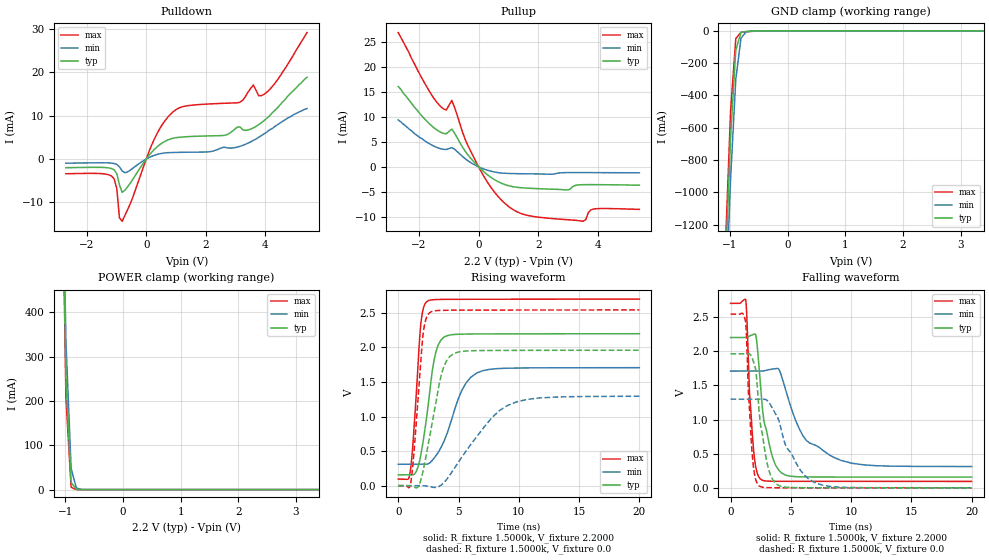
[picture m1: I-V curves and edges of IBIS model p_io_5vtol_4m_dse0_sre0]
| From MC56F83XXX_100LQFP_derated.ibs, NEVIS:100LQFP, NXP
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[Model] p_io_5vtol_4m_dse0_sre0
|   Model p_io_5vtol_4m_dse0_sre0
| Library cells for typ/min/max conditions are connected as defined below:
|  pad - External Pad
|  ipp_do - Core Input
|  ipp_obe - Output Buffer Enable
|  esd_boost - vdd_s_3v
|  esd_bus - vdd_s_3v
|  ipp_ame - vss_s_lv
|  ipp_dse - vss_s_lv
|  ipp_ina40a_5vtol - NC
|  ipp_ina40b_5vtol - NC
|  ipp_ina_5vtol - NC
|  ipp_ina_mux_3v - NC
|  ipp_ind - NC
|  ipp_ind_3v - NC
|  ipp_pue - vss_s_lv
|  ipp_sre - vss_s_lv
|  tie_3v - vdd_s_3v
|  tie_hi - vdd_s_lv
|  vbuf_3v - vdd_s_3v
|  vdd_bulk_lv - vdd_s_lv
|  vdd_s_3v - vdd_s_3v
|  vdd_s_lv - vdd_s_lv
|  vss_bulk - vss_s_3v
|  vss_s_3v - vss_s_3v
|  vss_s_lv - vss_s_lv
| All other pins connected to ground
Model_type I/O
Polarity   Non-Inverting
Enable   Active-High
Vinl =   0.7700V
Vinh =   1.5400V
Vmeas =  1.1000V
Cref =   25.0000pF
Rref =   1.0000k
Vref =   0.0V
C_comp   2.5897pF   2.5141pF   2.6932pF
[Temperature Range]   25.0000   0.1250k   -40.0000
[Voltage Range]   2.2000V   1.7100V   2.7000V
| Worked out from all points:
|   slope of the pulldown table from 0 to 0.33 V, typ, clamps not added: 128 ohm
|   slope of the pullup table from 0 to 0.33 V, typ, clamps not added: 190 ohm
|   GND clamp passes 1 mA (typ) near -0.56 V on its own axis
|   POWER clamp passes 1 mA (typ) near -0.81 V on its own axis
|   rising waveform, R_fixture 1.5000k, V_fixture 2.2000: 20-80 % time 947ps typ, 1.78ns min, 566ps max; typ from 0.156 V to 2.2 V
|   rising waveform, R_fixture 1.5000k, V_fixture 0.0: 20-80 % time 1.26ns typ, 3.4ns min, 656ps max; typ from 0 V to 1.96 V
|   falling waveform, R_fixture 1.5000k, V_fixture 2.2000: 20-80 % time 953ps typ, 2.78ns min, 464ps max; typ from 2.2 V to 0.158 V
|   falling waveform, R_fixture 1.5000k, V_fixture 0.0: 20-80 % time 819ps typ, 1.91ns min, 430ps max; typ from 1.96 V to 0.001 V
[Pulldown]
|Voltage   I(typ)   I(min)   I(max)
-2.7V     -2mA       -960uA     -3.39mA
-1.17V    -2.19mA    -943uA     -3.913mA
-990mV    -3.359mA   -1.244mA   -6.804mA
-900mV    -5.941mA   -1.821mA   -13.58mA
-810mV    -7.677mA   -2.75mA    -14.34mA
270mV     2.201mA    843.7uA    4.568mA
810mV     4.605mA    1.475mA    10.28mA
3.15V     7.385mA    2.91mA     13.07mA
3.6V      7.17mA     4.3mA      17.03mA
3.78V     7.91mA     5mA        14.56mA
3.96V     8.86mA     5.8mA      14.91mA
5.4V      18.8mA     11.6mA     29.1mA
[Pullup]
|Voltage   I(typ)   I(min)   I(max)
-2.7V     16.1mA     9.4mA      26.9mA
-1.44V    7.55mA     3.98mA     13.23mA
-1.08V    6.637mA    3.488mA    11.41mA
-900mV    7.558mA    3.848mA    13.31mA
-450mV    3.121mA    1.623mA    5.492mA
90mV      -525.5uA   -231.9uA   -998.2uA
540mV     -2.585mA   -1.04mA    -5.11mA
1.08V     -3.888mA   -1.337mA   -8.259mA
2.97V     -4.634mA   -1.154mA   -10.59mA
3.51V     -3.575mA   -1.148mA   -10.91mA
3.87V     -3.565mA   -1.16mA    -8.446mA
5.4V      -3.68mA    -1.2mA     -8.52mA
[GND_clamp]
|Voltage   I(typ)   I(min)   I(max)
-2.7V     -20.35A    -20.38A    -20.37A
-1.08V    -1.486A    -1.737A    -1.339A
-990mV    -654.8mA   -915.7mA   -496.6mA
-900mV    -120.3mA   -300.6mA   -47.98mA
-810mV    -10.43mA   -45.61mA   -9.206mA
-720mV    -3.577mA   -6.172mA   -6.342mA
-540mV    -682.6uA   -563.7uA   -1.265mA
5.4V      0A         0A         0A
[POWER_clamp]
|Voltage   I(typ)   I(min)   I(max)
-2.7V     20.23A     19.96A     20.45A
-1.08V    950.5mA    990.2mA    948mA
-990mV    252.7mA    333.8mA    206.6mA
-900mV    16.05mA    47.59mA    5.278mA
-810mV    508.3uA    3.841mA    61.17uA
-720mV    15.33uA    281.3uA    694.4nA
-630mV    461.8nA    20.43uA    7.955nA
5.4V      0A         0A         0A
[Ramp]
| variable   typ   min   max
dV/dt_r  0.1310/0.6099n   41.9192m/0.9827n   0.3059/0.4620n
dV/dt_f  0.1585/0.2908n   47.3400m/0.4162n   0.3794/0.2202n
R_load = 50.0000
[Rising Waveform]
R_fixture= 1.5000k
V_fixture= 2.2000
V_fixture_min= 1.7100
V_fixture_max= 2.7000
|time   V(typ)   V(min)   V(max)
0s        156.3mV    309.1mV    94.08mV
1.008ns   156.1mV    309mV      214.5mV
1.223ns   156.9mV    309.1mV    604.9mV
1.884ns   453.4mV    309.7mV    2.358V
2.357ns   988.2mV    310.8mV    2.661V
3.11ns    1.925V     428.6mV    2.692V
4.041ns   2.17V      748mV      2.696V
5.622ns   2.194V     1.484V     2.697V
7.005ns   2.196V     1.663V     2.697V
20ns      2.198V     1.707V     2.699V
[Rising Waveform]
R_fixture= 1.5000k
V_fixture= 0.0
V_fixture_min= 0.0
V_fixture_max= 0.0
|time   V(typ)   V(min)   V(max)
0s        2.604nV    511.6nV    74.27pV
1.045ns   -1.902mV   -16.32uV   46.18mV
1.637ns   -19.77mV   562.3uV    1.241V
2.067ns   214.7mV    -137.8uV   2.196V
2.59ns    691.2mV    -13.1mV    2.501V
3.57ns    1.602V     7.719mV    2.537V
4.581ns   1.908V     230.7mV    2.539V
7.764ns   1.956V     982.8mV    2.541V
9.789ns   1.957V     1.211V     2.541V
20ns      1.959V     1.293V     2.542V
[Falling Waveform]
R_fixture= 1.5000k
V_fixture= 2.2000
V_fixture_min= 1.7100
V_fixture_max= 2.7000
|time   V(typ)   V(min)   V(max)
0s        2.2V       1.71V      2.7V
1.266ns   2.199V     1.71V      2.746V
1.857ns   2.244V     1.71V      666.2mV
2.139ns   2.193V     1.71V      267.4mV
2.491ns   1.482V     1.709V     127.5mV
3.471ns   456.6mV    1.739V     97.48mV
4.547ns   189.1mV    1.449V     96.53mV
6.025ns   161.2mV    756.7mV    96.23mV
8.664ns   159.3mV    438.4mV    95.93mV
20ns      158mV      313.1mV    95.07mV
[Falling Waveform]
R_fixture= 1.5000k
V_fixture= 0.0
V_fixture_min= 0.0
V_fixture_max= 0.0
|time   V(typ)   V(min)   V(max)
0s        1.962V     1.3V       2.544V
1.23ns    1.961V     1.299V     2.448V
1.507ns   1.965V     1.299V     1.307V
1.821ns   1.888V     1.299V     441mV
2.08ns    1.736V     1.299V     125.6mV
2.34ns    1.185V     1.299V     33.41mV
3.172ns   261.8mV    1.254V     3.37mV
4.045ns   30.97mV    963.9mV    2.355mV
7.029ns   2.701mV    73.09mV    1.814mV
20ns      1.37mV     2.257mV    877.9uV
